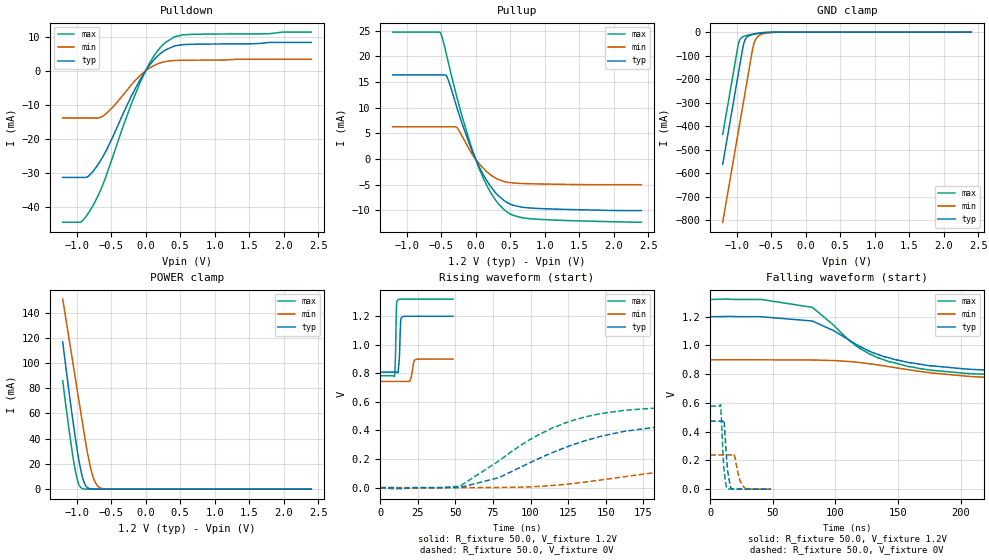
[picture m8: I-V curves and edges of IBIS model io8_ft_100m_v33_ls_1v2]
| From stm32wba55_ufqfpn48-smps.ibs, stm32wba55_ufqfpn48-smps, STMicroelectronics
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[Model]   io8_ft_100m_v33_ls_1v2
Model_type I/O
Polarity   Non-Inverting
Enable   Active-Low
| CAP_THRESHOLD on pad IOFT is "UDTCAPC" :
| Rising=30.0% of vddiom   Falling=70.0% of vddiom
| C_comp min and max val. don't necessarily correlate with the min and max pvt
| but are the smallest and greatest pad capacitance found.
| var   typ   min   max
C_comp   1.83455pF  1.64921pF  1.97628pF
|C_comp_pullup   1.12475pF  1.02555pF  1.16070pF
|C_comp_pulldown   709.80000fF  623.66501fF  815.58000fF
Vinl = 450.0mV
Vinh = 660.0mV
Vmeas = 600.0mV   | Reference voltage for timing measurements
Cref  = 50.0pF   | Timing specification test load capacitance value
Rref  = 1.0MOhm   | Timing specification test load resistance value
Vref  = 660.0mV   | Timing specification test load voltage
[Model Spec]
| TIME_THRESHOLD on pin ZIV33M is "CMOS" :
| Rising=50.0% of vddiom   Falling=50.0% of vddiom
Vinl 436.50000mV 342.50000mV 466.50000mV
Vinh 753.50000mV 549.50000mV 839.50000mV
| variable   typ   min   max
[Temperature Range] 25.0 140.0 -40.0
| variable   typ   min   max
[Voltage Range] 1.2V 900.0mV 1.32V
| variable   typ   min   max
[POWER Clamp Reference] 1.2V 900.0mV 1.32V
| variable   typ   min   max
[GND Clamp Reference] 0V 0V 0V
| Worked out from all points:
|   slope of the pulldown table from 0 to 0.18 V, typ, clamps not added: 40.6 ohm
|   slope of the pullup table from 0 to 0.18 V, typ, clamps not added: 39.4 ohm
|   GND clamp passes 1 mA (typ) near -0.51 V on its own axis
|   POWER clamp passes 1 mA (typ) near -0.83 V on its own axis
|   rising waveform, R_fixture 50.0, V_fixture 1.2V: 20-80 % time 821ps typ, 1.54ns min, 596ps max; typ from 0.809 V to 1.2 V
|   falling waveform, R_fixture 50.0, V_fixture 1.2V: 20-80 % time 61.6ns typ, 97.4ns min, 52.8ns max; typ from 1.2 V to 0.809 V
|   rising waveform, R_fixture 50.0, V_fixture 0V: 20-80 % time 71.5ns typ, 124ns min, 57.4ns max; typ from 0 V to 0.473 V
|   falling waveform, R_fixture 50.0, V_fixture 0V: 20-80 % time 2.69ns typ, 4.08ns min, 2.22ns max; typ from 0.473 V to 0 V
[POWER Clamp]
-1.2V     116.7mA    150.7mA    85.92mA
-1.06V    57.23mA    102.6mA    28.68mA
-1.02V    41.75mA    88.91mA    15.5mA
-980mV    27.6mA     75.18mA    5.935mA
-920mV    10.75mA    54.6mA     597.6uA
-870mV    3.065mA    37.68mA    60.82uA
-820mV    594.6uA    22.85mA    5.912uA
-770mV    99.71uA    11.47mA    572nA
-730mV    23.34uA    5.552mA    88.29nA
-680mV    3.779uA    1.833mA    8.565nA
-510mV    7.889nA    23.13uA    53.67pA
2.4V      0A         0A         0A
[GND Clamp]
-1.2V     -561.6mA   -807.5mA   -434.8mA
-980mV    -187.6mA   -433.5mA   -60.76mA
-960mV    -153.6mA   -399.5mA   -38.21mA
-900mV    -54.17mA   -297.5mA   -18.87mA
-870mV    -29.55mA   -246.5mA   -15.73mA
-830mV    -17.05mA   -178.5mA   -12.57mA
-760mV    -9.921mA   -62.77mA   -8.045mA
-730mV    -8.191mA   -35.56mA   -6.403mA
-680mV    -5.826mA   -15.57mA   -4.089mA
-580mV    -2.43mA    -5.043mA   -1.157mA
-330mV    -11.72uA   -245.5uA   -300.5nA
2.4V      872pA      1.055uA    338.3pA
| variable   typ   min   max
[Pullup Reference] 1.2V 900.0mV 1.32V
| variable   typ   min   max
[Pulldown Reference] 0V 0V 0V
[Pullup]
-1.2V     16.39mA    6.277mA    24.72mA
-510mV    16.39mA    6.277mA    24.58mA
-470mV    16.39mA    6.277mA    23.01mA
-410mV    15.89mA    6.277mA    19.68mA
-270mV    10mA       6.109mA    12.02mA
-80mV     2.58mA     1.624mA    3.14mA
10mV      -297.9uA   -180.5uA   -364.9uA
120mV     -3.232mA   -1.915mA   -3.953mA
230mV     -5.55mA    -3.196mA   -6.777mA
450mV     -8.417mA   -4.493mA   -10.26mA
790mV     -9.528mA   -4.811mA   -11.62mA
2.4V      -10.04mA   -4.994mA   -12.3mA
[Pulldown]
-1.2V     -31.2mA    -13.81mA   -44.3mA
-940mV    -31.2mA    -13.81mA   -44.26mA
-850mV    -31.11mA   -13.81mA   -42.26mA
-760mV    -29.39mA   -13.81mA   -39.38mA
-660mV    -26.52mA   -13.68mA   -35.32mA
-560mV    -22.95mA   -12.35mA   -30.17mA
-330mV    -12.74mA   -7.204mA   -16.5mA
-80mV     -2.622mA   -1.37mA    -3.49mA
100mV     2.727mA    1.319mA    3.679mA
290mV     6.144mA    2.737mA    8.347mA
540mV     7.674mA    3.096mA    10.53mA
2.4V      8.319mA    3.393mA    11.34mA
[Ramp]
dV/dt_r 283.79555mV/70.94257ns 142.76467mV/123.48332ns 346.61973mV/55.64128ns
dV/dt_f 234.6596mV/60.34443ns 93.75834mV/93.19302ns 321.77283mV/51.61281ns
R_load = 50.0
| Removed startup time: 0s 0s 0s  .
| Removed end time: 48.4ns.
[Rising Waveform]
R_fixture   = 50.0
V_fixture   = 1.2V
V_fixture_min = 900.0mV
V_fixture_max = 1.32V
0s        808.9mV    743.7mV    783.7mV
9.45ns    808.9mV    743.7mV    780mV
10.1ns    809mV      743.7mV    914.7mV
10.8ns    808.4mV    743.7mV    1.274V
11.7ns    804.1mV    743.7mV    1.316V
12.65ns   897.9mV    743.7mV    1.319V
13.6ns    1.166V     743.7mV    1.319V
14.85ns   1.198V     743.7mV    1.32V
23.75ns   1.2V       897.8mV    1.32V
48.4ns    1.2V       899.9mV    1.32V
| Removed startup time: 0s 0s 0s  .
| Removed end time: 1.9984us.
[Falling Waveform]
R_fixture   = 50.0
V_fixture   = 1.2V
V_fixture_min = 900.0mV
V_fixture_max = 1.32V
0s        1.2V       900mV      1.32V
40.8ns    1.2V       900.1mV    1.32V
81.55ns   1.17V      898.9mV    1.265V
116.5ns   1.008V     883.8mV    996.3mV
128ns     957mV      871.6mV    936.6mV
143.3ns   912.3mV    851.7mV    884.9mV
176.4ns   858.8mV    809.3mV    827.8mV
244.7ns   820.1mV    767.7mV    792mV
489.4ns   808.9mV    744.4mV    783.7mV
1.998us   808.9mV    743.7mV    783.7mV
| Removed startup time: 0s 0s 0s  .
| Removed end time: 1.9984us.
[Rising Waveform]
R_fixture   = 50.0
V_fixture   = 0V
V_fixture_min = 0V
V_fixture_max = 0V
0s        4.84nV     985.4nV    4.251nV
53ns      1.227mV    55.91uV    10.01mV
78.7ns    69.22mV    1.224mV    185.3mV
100.6ns   179.7mV    5.554mV    343.4mV
123.7ns   282.8mV    23.65mV    455.9mV
163.2ns   395.2mV    77.53mV    541.9mV
203.9ns   444.1mV    133.5mV    567.7mV
285.5ns   469.1mV    201.3mV    577.2mV
423.9ns   473mV      233.2mV    577.8mV
1.998us   473mV      237.9mV    577.7mV
| Removed startup time: 0s 0s 0s  .
| Removed end time: 48.4ns.
[Falling Waveform]
R_fixture   = 50.0
V_fixture   = 0V
V_fixture_min = 0V
V_fixture_max = 0V
0s        473mV      238mV      577.7mV
8.25ns    473mV      238mV      587.6mV
10.95ns   478.8mV    238mV      137.9mV
13.2ns    195.5mV    238mV      6.002mV
14ns      119.4mV    238mV      2.283mV
16.8ns    5.298mV    238mV      662.5uV
18.95ns   1.118mV    242.8mV    270.9uV
23.7ns    193.9uV    60.47mV    110.4uV
27.3ns    97.59uV    10.02mV    92.73uV
48.4ns    85.76uV    51.31uV    92.11uV
